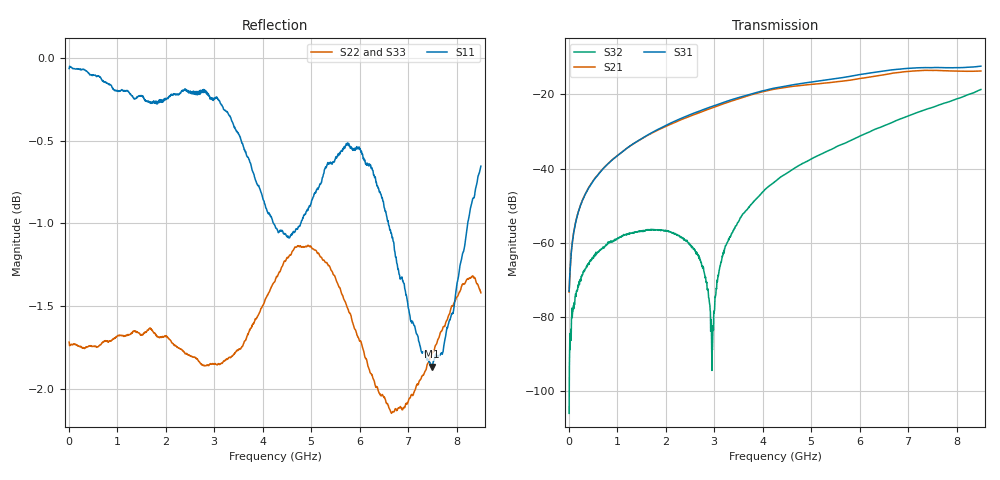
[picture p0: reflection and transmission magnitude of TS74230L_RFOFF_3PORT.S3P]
!Agilent Technologies,E5071C,MY46522130,B.12.04
!Date: Wed Jul 30 10:25:43 2025
!Data & Calibration Information:
!Freq	S11:SOLT3(ON)	S13:SOLT3(ON)	S14:SOLT3(ON)
!	S31:SOLT3(ON)	S33:SOLT3(ON)	S34:SOLT3(ON)
!	S41:SOLT3(ON)	S43:SOLT3(ON)	S44:SOLT3(ON)
!PortZ  Port1:50+j0  Port3:50+j0  Port4:50+j0
!Above PortZ is port z conversion or system Z0 setting when saving the data.
!When reading, reference impedance value at option line is always used.
# Hz S dB R 50
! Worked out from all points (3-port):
!   1601 points, 10 MHz to 8.5 GHz, reference 50 ohm
!   strongest paths, dB at 10 MHz, 2.132 GHz, 4.255 GHz, 6.378 GHz, 8.5 GHz:
!     S31: -73.0, -27.5, -18.3, -13.9, -12.4
!     S21: -73.3, -27.9, -18.6, -15.0, -13.7
!     S32: -105.9, -57.3, -43.5, -29.1, -18.7
!   lowest |S11| = -1.9 dB at 7.487 GHz (marker M1), VSWR 9.35, Z = 6.71 + j25 ohm
!   |S11| at or under -10 dB: nowhere
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1e7  -0.07 -0.2  -73.46 44.5  -74.24 40.4
     -73.27 43.8  -1.72 179.4  -100.45 145.1
     -73.01 40.5  -105.90 -107.8  -1.70 179.4
3.814375e8  -0.08 -9.3  -45.83 90.6  -45.97 91.1
            -45.80 90.6  -1.75 170.5  -65.92 82.3
            -45.95 91.3  -65.99 81.1  -1.72 170.5
1.681469e9  -0.27 -48.7  -30.65 89.1  -30.55 91.2
            -30.67 89.0  -1.63 141.9  -56.37 61.9
            -30.55 91.1  -56.52 61.5  -1.64 144.0
2.610062e9  -0.22 -73.0  -25.31 78.9  -24.89 79.9
            -25.32 78.7  -1.81 122.1  -61.94 41.4
            -24.90 79.8  -62.30 43.5  -1.93 121.5
2.965581e9  -0.25 -80.7  -23.59 74.2  -23.20 74.6
            -23.60 74.1  -1.85 113.6  -88.03 -114.9
            -23.21 74.6  -88.80 -72.3  -1.93 111.7
3.268038e9  -0.33 -88.1  -22.19 69.3  -21.81 69.5
            -22.19 69.2  -1.82 106.7  -60.02 -147.5
            -21.82 69.4  -59.95 -148.0  -1.87 104.1
4.255e9  -1.01 -128.0  -18.55 46.7  -18.27 48.1
         -18.56 46.5  -1.35 87.4  -43.55 -170.8
         -18.28 47.9  -43.46 -170.6  -1.30 88.2
5.974225e9  -0.55 178.3  -15.80 14.7  -14.72 14.6
            -15.78 14.8  -1.69 68.1  -31.38 150.5
            -14.72 14.7  -31.43 150.4  -2.00 66.6
7.486506e9  -1.87 126.1  -13.53 -19.3  -12.79 -21.3
            -13.55 -19.7  -1.79 36.8  -23.44 117.4
            -12.80 -21.5  -23.57 117.7  -1.73 31.8
8.5e9  -0.65 98.3  -13.69 -35.0  -12.40 -35.7
       -13.70 -35.3  -1.42 27.9  -18.78 96.2
       -12.39 -36.0  -18.68 96.8  -1.59 29.5
